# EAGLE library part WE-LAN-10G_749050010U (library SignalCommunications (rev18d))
WE-LAN 10G Transformer 10Gbit Base-T - Compliant with standards: IEEE 802.3an and upcoming IEEE 802.3bt - SMD -- Ethernet -- Ethernet speed up to 10Gbit/s --Power over Ethernet PoE and PoE+ --10Gbit with ETR and PoE up to 150 W (for industrial applications) Details see: http://katalog.we-online.de/en/pbs/WE-LAN-10G 2016 (C) Würth Elektronik
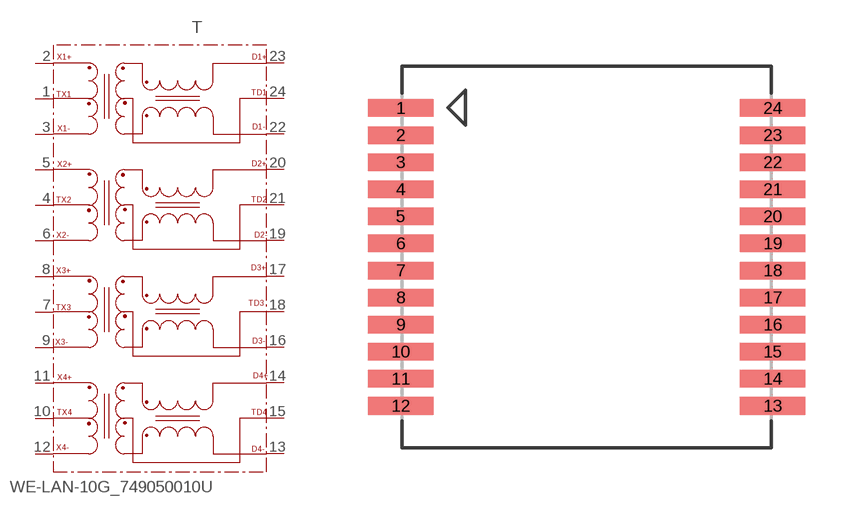
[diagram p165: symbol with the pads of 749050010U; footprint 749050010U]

Designator prefix T

## WE-LAN-10G_749050010U  [749050010U]
1  TX1
2  X1+
3  X1-
4  TX2
5  X2+
6  X2-
7  TX3
8  X3+
9  X3-
10  TX4
11  X4+
12  X4-
13  D4-
14  D4+
15  TD4
16  D3-
17  D3+
18  TD3
19  D2-
20  D2+
21  TD2
22  D1-
23  D1+
24  TD1

## Footprint 749050010U (pad centres in mm)
smd 2.4 x 0.64: 1 -6.8,5.445; 2 -6.8,4.455; 3 -6.8,3.465; 4 -6.8,2.475; 5 -6.8,1.485; 6 -6.8,0.495; 7 -6.8,-0.495; 8 -6.8,-1.485; 9 -6.8,-2.475; 10 -6.8,-3.465; 11 -6.8,-4.455; 12 -6.8,-5.445; 13 6.8,-5.445; 14 6.8,-4.455; 15 6.8,-3.465; 16 6.8,-2.475; 17 6.8,-1.485; 18 6.8,-0.495; 19 6.8,0.495; 20 6.8,1.485; 21 6.8,2.475; 22 6.8,3.465; 23 6.8,4.455; 24 6.8,5.445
